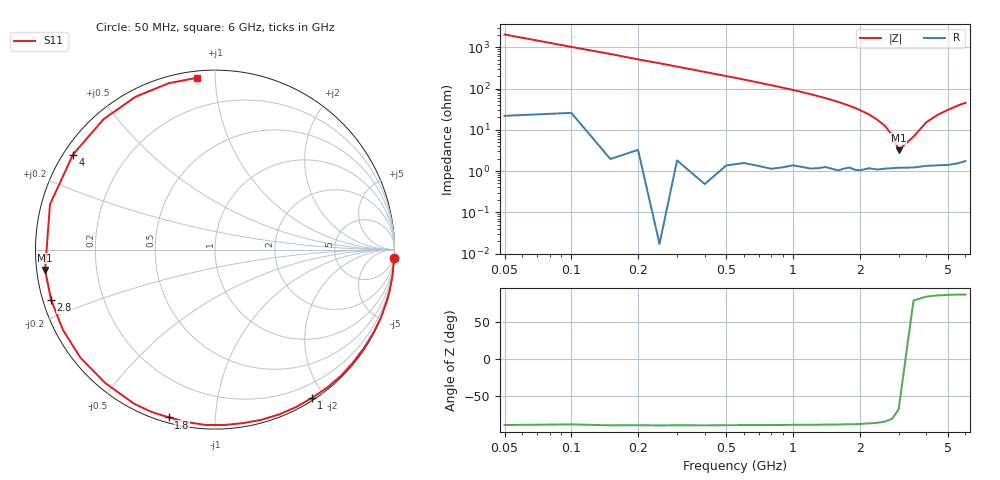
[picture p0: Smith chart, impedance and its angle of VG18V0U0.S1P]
! Infineon Technologies  Discrete & RF Semiconductors
! BB 831
! Si Tuning Diode in SOD323
! VR = 18 V
! S-Parameters:  July  1999
# GHz  S  MA  R  50
!  f  S11
! GHz  MAG  ANG
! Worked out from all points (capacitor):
!   34 points, 50 MHz to 6 GHz, reference 50 ohm
!   read as one part to ground: C = 1.56 pF near 50 MHz
!   lowest |Z| = 3.2 ohm at 3 GHz (marker M1)
!   series resonance near 3.153 GHz, so ESL is about 1.6 nH
!   S11 on the Smith chart (normalised r, x): 50 MHz: 0, -41; 1 GHz: 0.03, -1.85; 1.8 GHz: 0.02, -0.76; 2.8 GHz: 0.02, -0.15; 4 GHz: 0.03, +0.30; 6 GHz: 0.03, +0.90
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0.05  0.9995 -2.8
0.15  0.9996 -8.3
0.25  1 -13.9
0.4  0.9993 -22.4
0.6  0.9948 -33.6
0.8  0.9933 -45.2
0.9  0.9909 -51.0
1  0.9876 -56.9
1.1  0.9865 -62.8
1.2  0.9854 -68.8
1.3  0.9828 -74.9
1.5  0.9787 -86.9
1.6  0.9784 -93.1
1.7  0.9737 -99.4
1.8  0.9697 -105.4
1.9  0.9711 -111.4
2  0.9699 -117.6
2.2  0.9626 -129.5
2.4  0.9619 -141.3
2.6  0.958 -152.2
2.8  0.9551 -163.0
3  0.9533 -173.2
3.5  0.9533 164.7
4  0.9523 146.2
4.5  0.9557 130.5
5  0.9597 117.5
5.5  0.9622 105.5
6  0.9622 96.0
